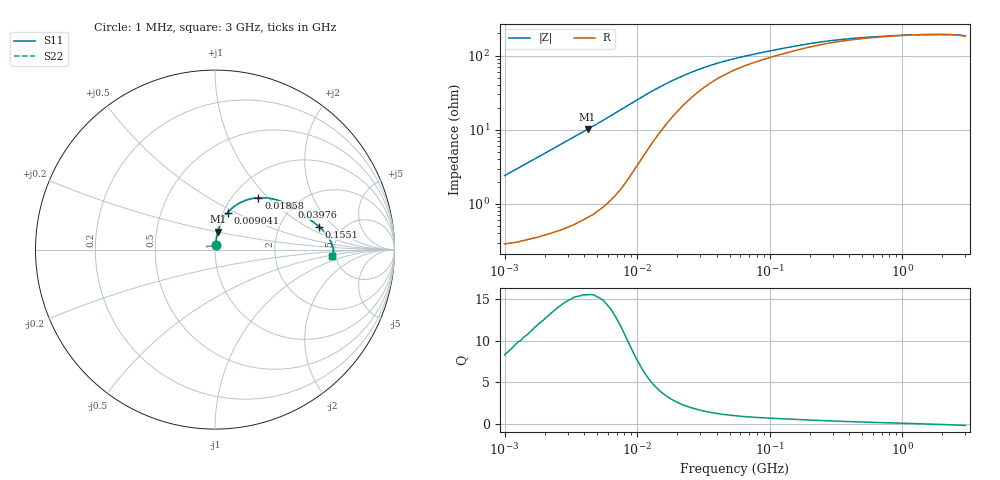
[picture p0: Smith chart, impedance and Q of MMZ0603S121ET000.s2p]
! S-Parameter Data Generated by TDK Corporation
! Copyright(C) 2025 TDK Corporation.
! All Rights Reserved.
! TDK P/N: MMZ0603S121ET000 (Chip Bead)
! Property: |Z|=120ohm at 100MHz
! Size(LxWxT): 0.6x0.3x0.3mm
! Model Type: s2p (Touchstone File Format Version 1.0)
! Frequency: DC=Yes Start=1MHz Stop=3000MHz 202points Log-sweep
! Model Generated on Feb. 6, 2025
! Terms and conditions regarding TDK Simulation Models:
! 1)This simulation model is being provided solely for informational
!  purposes. Please refer to the specifications of the products in
!  terms of detailed characteristics of such products.
! 2)In no event shall TDK Corporation of any of its subsidiaries be
!  liable for any loss or damage arising, directly or indirectly,
!  from any information contained in this simulation model, including,
!  but not limited to loss or damages arising from any inaccuracies,
!  omissions or errors in connection with such information.
! 3)Any and all copyrights on this simulation model are owned by
!  TDK Corporation.  Duplication or redistribution of this simulation
!  model without prior written permission from TDK Corporation
!  is prohibited.
! 4)This simulation model is subject to any modification or change
!  without any prior notice.
! 5)Neither TDK Corporation nor any of its subsidiaries shall make any
!  warranty, express or implied, including but not limited to the
!  correctness, implied warranties of merchantability and fitness for
!  a particular purpose with respect to this simulation models.
! 6)The use of this simulation model shall be deemed to have consented
!  to the terms and conditions hereof.
! Port Assignments:
!  1 ---@@@--- 2
! Applicable Conditions:
!  Temperature = 25 degC
!  DC Bias Current = 0 A
!  Small Signal Operation
# Hz S MA R 50
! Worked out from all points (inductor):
!   201 points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, 1 MHz to 3 GHz, reference 50 ohm
!   read as one part in series: L = 380 nH near 1.041 MHz
!   highest Q = 15.5 at 4.226 MHz (marker M1), where L = 382 nH
!   self-resonance near 1.664 GHz
!   S11 on the Smith chart (normalised r, x): 1 MHz: 1.01, +0.05; 9.041 MHz: 1.05, +0.45; 18.58 MHz: 1.30, +0.88; 39.76 MHz: 1.97, +1.24; 155.1 MHz: 3.35, +1.33; 3 GHz: 4.68, -0.59
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1000000  0.02401 81.8  0.9968 -1.4  0.9968 -1.4  0.02401 81.8
2139570  0.05095 82.7  0.9948 -2.9  0.9948 -2.9  0.05095 82.7
3900413  0.09278 81.0  0.9897 -5.3  0.9897 -5.3  0.09278 81.0
4225536  0.1005 80.6  0.9885 -5.8  0.9885 -5.8  0.1005 80.6
6563319  0.1573 76.7  0.9759 -9.0  0.9759 -9.0  0.1573 76.7
9040831  0.2175 71.2  0.9525 -12.5  0.9525 -12.5  0.2175 71.2
1.149534e7  0.271 65.1  0.9194 -15.5  0.9194 -15.5  0.271 65.1
1.461624e7  0.3257 57.8  0.8711 -18.4  0.8711 -18.4  0.3257 57.8
1.858443e7  0.3767 50.1  0.8114 -20.9  0.8114 -20.9  0.3767 50.1
2.181181e7  0.4068 45.1  0.7686 -22.0  0.7686 -22.0  0.4068 45.1
2.664524e7  0.4393 39.2  0.7155 -22.8  0.7155 -22.8  0.4393 39.2
3.254976e7  0.4666 33.9  0.666 -23.0  0.666 -23.0  0.4666 33.9
3.976269e7  0.4891 29.4  0.6221 -22.7  0.6221 -22.7  0.4891 29.4
5.477226e7  0.5184 23.6  0.5647 -21.6  0.5647 -21.6  0.5184 23.6
8.854986e7  0.5549 17.6  0.5 -19.6  0.5 -19.6  0.5549 17.6
1.550909e8  0.5932 12.5  0.4401 -17.0  0.4401 -17.0  0.5932 12.5
2.136344e8  0.6115 10.1  0.4121 -15.1  0.4121 -15.1  0.6115 10.1
3.894533e8  0.6349 6.3  0.3754 -10.7  0.3754 -10.7  0.6349 6.3
8.005644e8  0.6511 3.0  0.3514 -5.6  0.3514 -5.6  0.6511 3.0
1.855641e9  0.6595 -0.5  0.3406 0.9  0.3406 0.9  0.6595 -0.5
2.359433e9  0.6589 -1.7  0.3419 3.2  0.3419 3.2  0.6589 -1.7
3e9  0.6525 -3.2  0.3504 6.0  0.3504 6.0  0.6525 -3.2
